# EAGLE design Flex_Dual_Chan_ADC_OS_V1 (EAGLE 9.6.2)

## Sheet 1 of 3: ADC, FE, and Vref
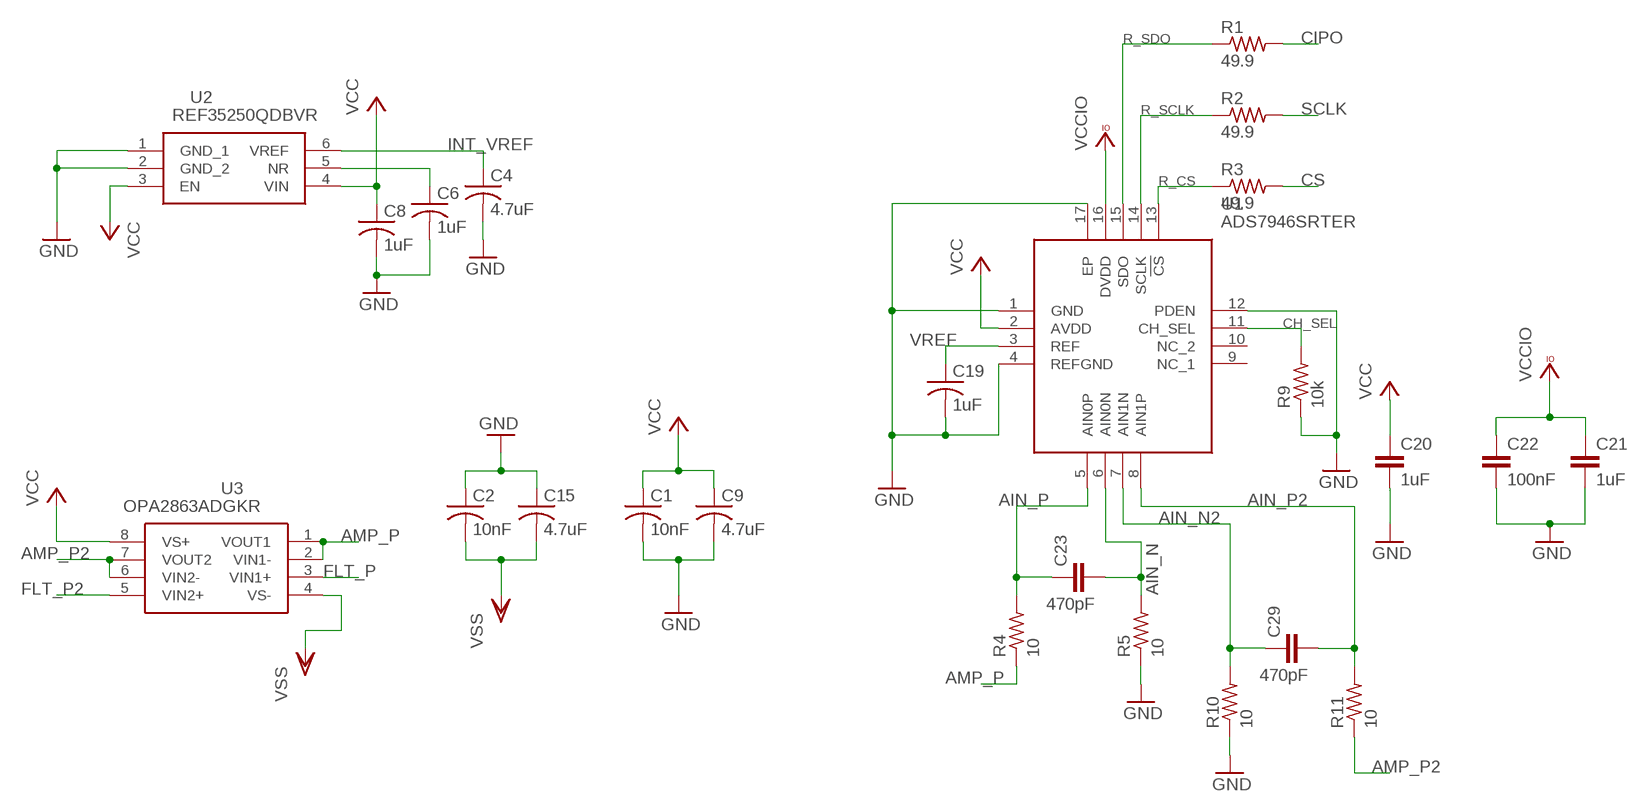
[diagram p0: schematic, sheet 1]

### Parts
C1  10nF  C-USC0603  [C0603]
C2  10nF  C-USC0603  [C0603]
C4  4.7uF  C-USC0603  [C0603]
C6  1uF  C-USC0603  [C0603]
C8  1uF  C-USC0603  [C0603]
C9  4.7uF  C-USC0603  [C0603]
C15  4.7uF  C-USC0603  [C0603]
C19  1uF  C-USC0603  [C0603]
C20  1uF  C-EUC0603  [C0603]
C21  1uF  C-EUC0603  [C0603]
C22  100nF  C-EUC0603  [C0603]
C23  470pF  C-EUC0603  [C0603]
C29  470pF  C-EUC0603  [C0603]
R1  49.9  R-US_R0603  [R0603]
R2  49.9  R-US_R0603  [R0603]
R3  49.9  R-US_R0603  [R0603]
R4  10  R-US_R0603  [R0603]
R5  10  R-US_R0603  [R0603]
R9  10k  R-US_R0603  [R0603]
R10  10  R-US_R0603  [R0603]
R11  10  R-US_R0603  [R0603]
U1  ADS7946SRTER  [QFN50P300X300X80-17N]
U2  REF35250QDBVR  REF35205QDBVR  [SOT95P280X145-6N]
U3  OPA2863ADGKR  [SOP65P490X110-8N]

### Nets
AIN_N: C23.2 R5.2 U1.6(AIN0N)
AIN_N2: C29.1 R10.2 U1.7(AIN1N)
AIN_P: C23.1 R4.2 U1.5(AIN0P)
AIN_P2: C29.2 R11.2 U1.8(AIN1P)
AMP_P: R4.1 U3.1(VOUT1) U3.2(VIN1-)
AMP_P2: R11.1 U3.6(VIN2-) U3.7(VOUT2)
CH_SEL: R9.2 U1.11(CH_SEL) ; also sheet 3
CIPO: R1.2 ; also sheet 3
CS: R3.2 ; also sheet 3
FLT_P: U3.3(VIN1+) ; also sheet 3
FLT_P2: U3.5(VIN2+) ; also sheet 3
GND: C1.2 C2.1 C4.2 C6.2 C8.2 C9.2 C15.1 C19.2 C20.2 C21.2 C22.2 R5.1 R9.1 R10.1 U1.1(GND) U1.4(REFGND) U1.12(PDEN) U1.17(EP) U2.1(GND_1) U2.2(GND_2) ; also sheet 2,3
INT_VREF: C4.1 U2.6(VREF) ; also sheet 2
N$2: C6.1 U2.5(NR)
R_CS: R3.1 U1.13(!CS)
R_SCLK: R2.1 U1.14(SCLK)
R_SDO: R1.1 U1.15(SDO)
SCLK: R2.2 ; also sheet 3
VCC: C1.1 C8.1 C9.1 C20.1 U1.2(AVDD) U2.3(EN) U2.4(VIN) U3.8(VS+) ; also sheet 2
VCCIO: C21.1 C22.1 U1.16(DVDD) ; also sheet 2
VREF: C19.1 U1.3(REF) ; also sheet 2,3
VSS: C2.2 C15.2 U3.4(VS-) ; also sheet 2
Unconnected: U1.9(NC_1) U1.10(NC_2)

## Sheet 2 of 3: Power Circuits
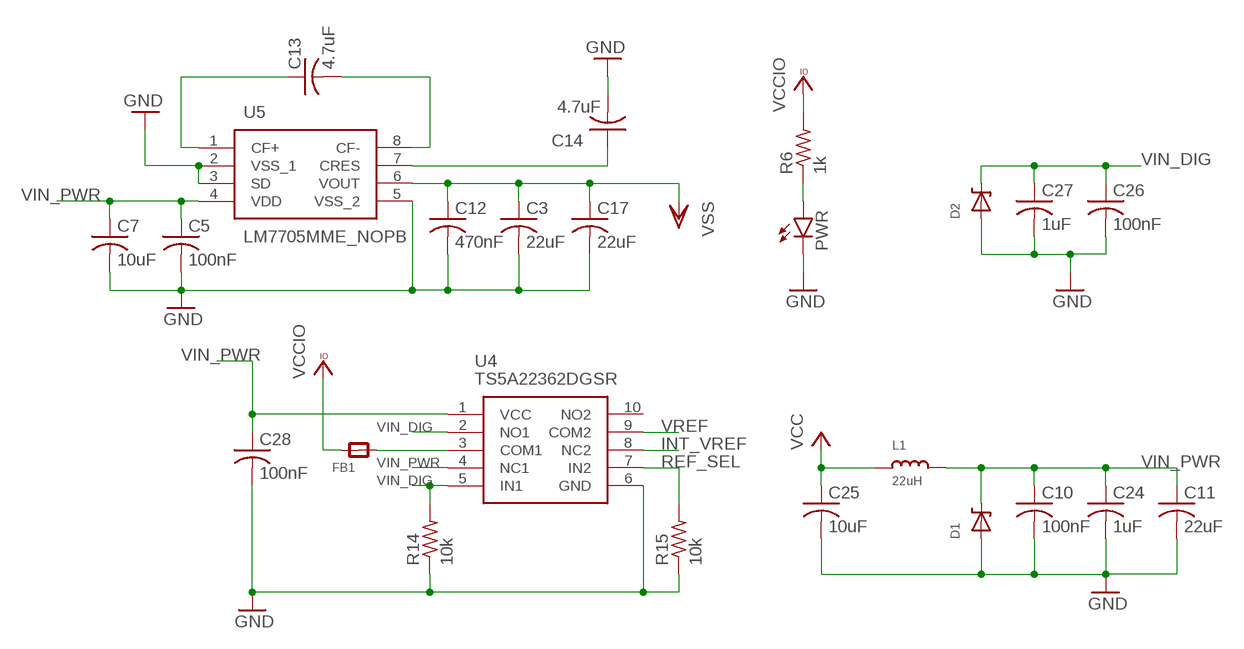
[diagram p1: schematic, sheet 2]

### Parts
C3  22uF  C-USC0603  [C0603]
C5  100nF  C-USC0603  [C0603]
C7  10uF  C-USC0603  [C0603]
C10  100nF  C-USC0603  [C0603]
C11  22uF  C-USC0603  [C0603]
C12  470nF  C-USC0603  [C0603]
C13  4.7uF  C-USC0603  [C0603]
C14  4.7uF  C-USC0603  [C0603]
C17  22uF  C-USC0603  [C0603]
C24  1uF  C-USC0603  [C0603]
C25  10uF  C-USC0603  [C0603]
C26  100nF  C-USC0603  [C0603]
C27  1uF  C-USC0603  [C0603]
C28  100nF  C-USC0603  [C0603]
D1  DDZ5V6ASF  [DDZ5V6ASF]
D2  DDZ5V6ASF  [DDZ5V6ASF]
FB1  FERRITE_0603  [_0603]
L1  22uH  INDUCTOR0805  [0805]
PWR  LEDCHIP-LED0603  [CHIP-LED0603]
R6  1k  R-US_R0603  [R0603]
R14  10k  R-US_R0603  [R0603]
R15  10k  R-US_R0603  [R0603]
U4  TS5A22362DGSR  [SOP50P490X110-10N]
U5  LM7705MME_NOPB  [SOP65P490X110-8N]

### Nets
GND: C3.2 C5.2 C7.2 C10.2 C11.2 C12.2 C14.2 C17.2 C24.2 C25.2 C26.2 C27.2 C28.2 D1.P$1(A) D2.P$1(A) PWR.C R14.1 R15.1 U4.6(GND) U5.2(VSS_1) U5.3(SD) U5.5(VSS_2) ; also sheet 1,3
INT_VREF: U4.8(NC2) ; also sheet 1
N$3: C13.1 U5.1(CF+)
N$4: PWR.A R6.1
N$5: C13.2 U5.8(CF-)
N$6: C14.1 U5.7(CRES)
N$7: FB1.2 U4.3(COM1)
REF_SEL: R15.2 U4.7(IN2)
VCC: C25.1 L1.1 ; also sheet 1
VCCIO: FB1.1 R6.2 ; also sheet 1
VIN_DIG: C26.1 C27.1 D2.P$2(C) R14.2 U4.2(NO1) U4.5(IN1) ; also sheet 3
VIN_PWR: C5.1 C7.1 C10.1 C11.1 C24.1 C28.1 D1.P$2(C) L1.2 U4.1(VCC) U4.4(NC1) U5.4(VDD) ; also sheet 3
VREF: U4.9(COM2) ; also sheet 1,3
VSS: C3.1 C12.1 C17.1 U5.6(VOUT) ; also sheet 1
Unconnected: U4.10(NO2)

## Sheet 3 of 3: Input Filter and Connections
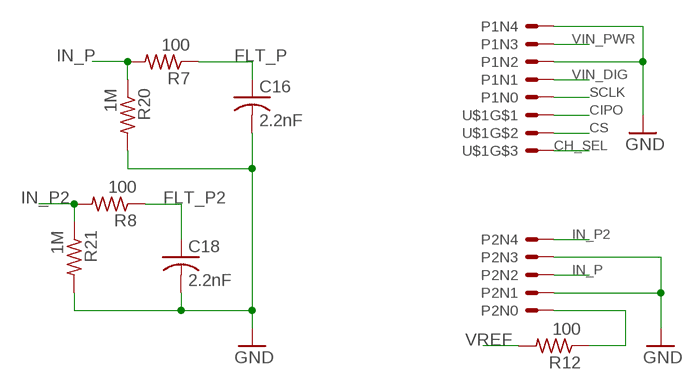
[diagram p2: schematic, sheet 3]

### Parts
C16  2.2nF  C-USC0603  [C0603]
C18  2.2nF  C-USC0603  [C0603]
P1  5PINHEADER  [5PINHEADER]
P2  5PINHEADER  [5PINHEADER]
R7  100  R-US_R0603  [R0603]
R8  100  R-US_R0603  [R0603]
R12  100  R-US_R0603  [R0603]
R20  1M  R-US_R0603  [R0603]
R21  1M  R-US_R0603  [R0603]
U$1  3PINHEADER  [3PINHEADER]

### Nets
CH_SEL: U$1.N2 ; also sheet 1
CIPO: U$1.N0 ; also sheet 1
CS: U$1.N1 ; also sheet 1
FLT_P: C16.1 R7.1 ; also sheet 1
FLT_P2: C18.1 R8.1 ; also sheet 1
GND: C16.2 C18.2 P1.N2 P1.N4 P2.N1 P2.N3 R20.2 R21.2 ; also sheet 1,2
IN_P: P2.N2 R7.2 R20.1
IN_P2: P2.N4 R8.2 R21.1
N$1: P2.N0 R12.1
SCLK: P1.N0 ; also sheet 1
VIN_DIG: P1.N1 ; also sheet 2
VIN_PWR: P1.N3 ; also sheet 2
VREF: R12.2 ; also sheet 1,2

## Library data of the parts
C1-C19 C24-C28 = rcl:C-US: CAPACITOR, American symbol; SPICEPREFIX: C
C20-C23 C29 = rcl:C-EU: CAPACITOR, European symbol; SPICEPREFIX: C
D1 D2 = ForceTronics:DDZ5V6ASF: DDZ5V6ASF 5.42 Zener Diode
FB1 = microbuilder:FERRITE: Ferrite Bead
L1 = microbuilder:INDUCTOR: Inductors
P1 = ForceTronics:5PINHEADER
P2 = ForceTronics-ForceTronics:5PINHEADER
PWR = led:LED: LED
R1-R12 R14 R15 R20 R21 = rcl:R-US_: RESISTOR, American symbol; SPICEPREFIX: R
U1 = SamacSys_Parts:ADS7946SRTER: 14-Bit, 2MSPS, Dual-Channel, Unipolar, Pseudo-Differential, u-Power SAR ADC Source: Datasheet; DESCRIPTION: 14-Bit, 2MSPS, Dual-Channel, Unipolar, Pseudo-Differential, u-Power SAR ADC; HEIGHT: 0.8mm; MANUFACTURER_NAME: Texas Instruments; MANUFACTURER_PART_NUMBER: ADS7946SRTER; MOUSER_PART_NUMBER: 595-ADS7946SRTER; MOUSER_PRICE-STOCK: https://www.mouser.co.uk/ProductDetail/Texas-Instruments/ADS7946SRTER?qs=UlfnwZ2x8nQ8ZHHj9riOig%3D%3D
U2 = SamacSys_Parts:REF35205QDBVR: Voltage References 650-nA quiescent current, 12-ppm/C drift, ultra-low-power precision voltage reference Source: Datasheet; DESCRIPTION: Voltage References 650-nA quiescent current, 12-ppm/C drift, ultra-low-power precision voltage reference; HEIGHT: 1.45mm; MANUFACTURER_NAME: Texas Instruments; MANUFACTURER_PART_NUMBER: REF35205QDBVR; MOUSER_PART_NUMBER: 595-REF35205QDBVR; MOUSER_PRICE-STOCK: https://www.mouser.co.uk/ProductDetail/Texas-Instruments/REF35205QDBVR?qs=rQFj71Wb1eUmjih2GyUdJQ%3D%3D
U3 = SamacSys_Parts:OPA2863ADGKR: Precision Amplifiers Dual, high-precision, low-power, 105MHz, 12V RRIO voltage-feedback amplifier Source: Datasheet; DESCRIPTION: Precision Amplifiers Dual, high-precision, low-power, 105MHz, 12V RRIO voltage-feedback amplifier; HEIGHT: 1.1mm; MANUFACTURER_NAME: Texas Instruments; MANUFACTURER_PART_NUMBER: OPA2863ADGKR
U4 = SamacSys_Parts:TS5A22362DGSR: Texas Instruments TS5A22362DGSR, Analogue Switch Dual SPDT, 2.3 5.5 V, 10-Pin VSSOP Source: Datasheet; DESCRIPTION: Texas Instruments TS5A22362DGSR, Analogue Switch Dual SPDT, 2.3 5.5 V, 10-Pin VSSOP; HEIGHT: 1.1mm; MANUFACTURER_NAME: Texas Instruments; MANUFACTURER_PART_NUMBER: TS5A22362DGSR; MOUSER_PART_NUMBER: 595-TS5A22362DGSR; MOUSER_PRICE-STOCK: https://www.mouser.co.uk/ProductDetail/Texas-Instruments/TS5A22362DGSR?qs=snW7ThfrdqwrWVQhLBj0GQ%3D%3D
U5 = SamacSys_Parts:LM7705MME_NOPB: Texas Instruments LM7705MME/NOPB Inverter, 3 5.25 V, 8-Pin MSOP Source: Datasheet; DESCRIPTION: Texas Instruments LM7705MME/NOPB Inverter, 3 5.25 V, 8-Pin MSOP; HEIGHT: 1.1mm; MANUFACTURER_NAME: Texas Instruments; MANUFACTURER_PART_NUMBER: LM7705MME/NOPB; MOUSER_PART_NUMBER: 926-LM7705MME/NOPB; MOUSER_PRICE-STOCK: https://www.mouser.co.uk/ProductDetail/Texas-Instruments/LM7705MME-NOPB?qs=QbsRYf82W3FggmdQUdGwaQ%3D%3D
U$1 = ForceTronics:3PINHEADER: 3 pin header with oval copper

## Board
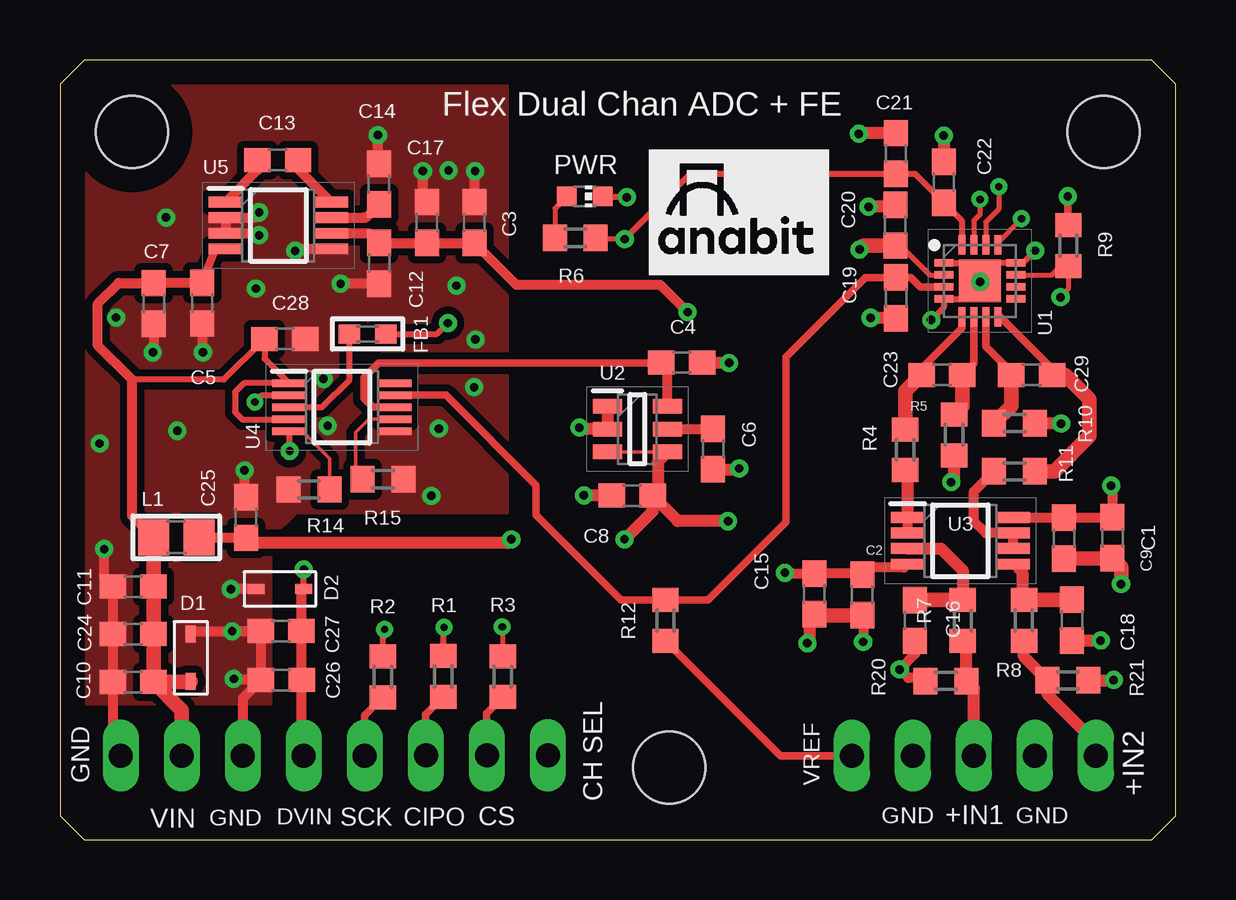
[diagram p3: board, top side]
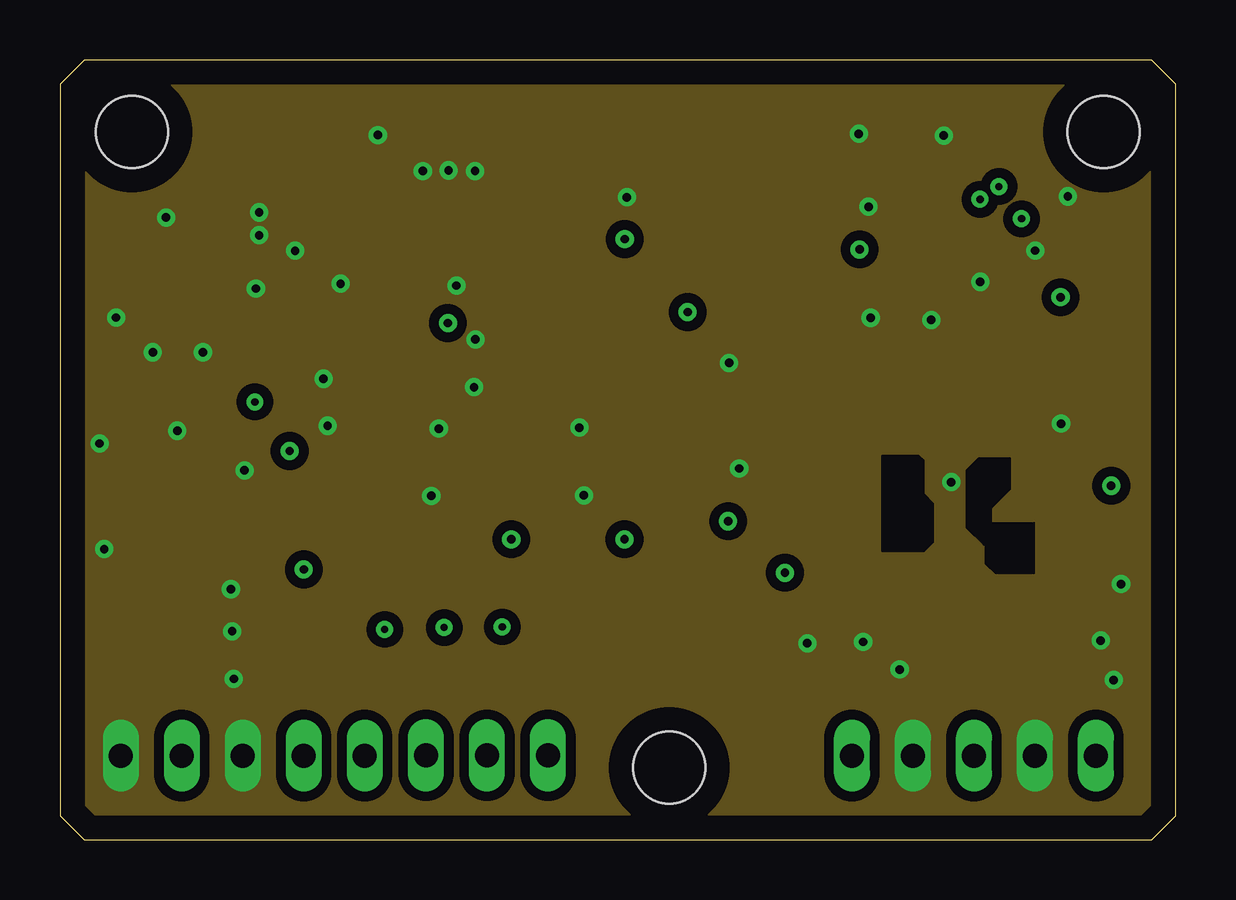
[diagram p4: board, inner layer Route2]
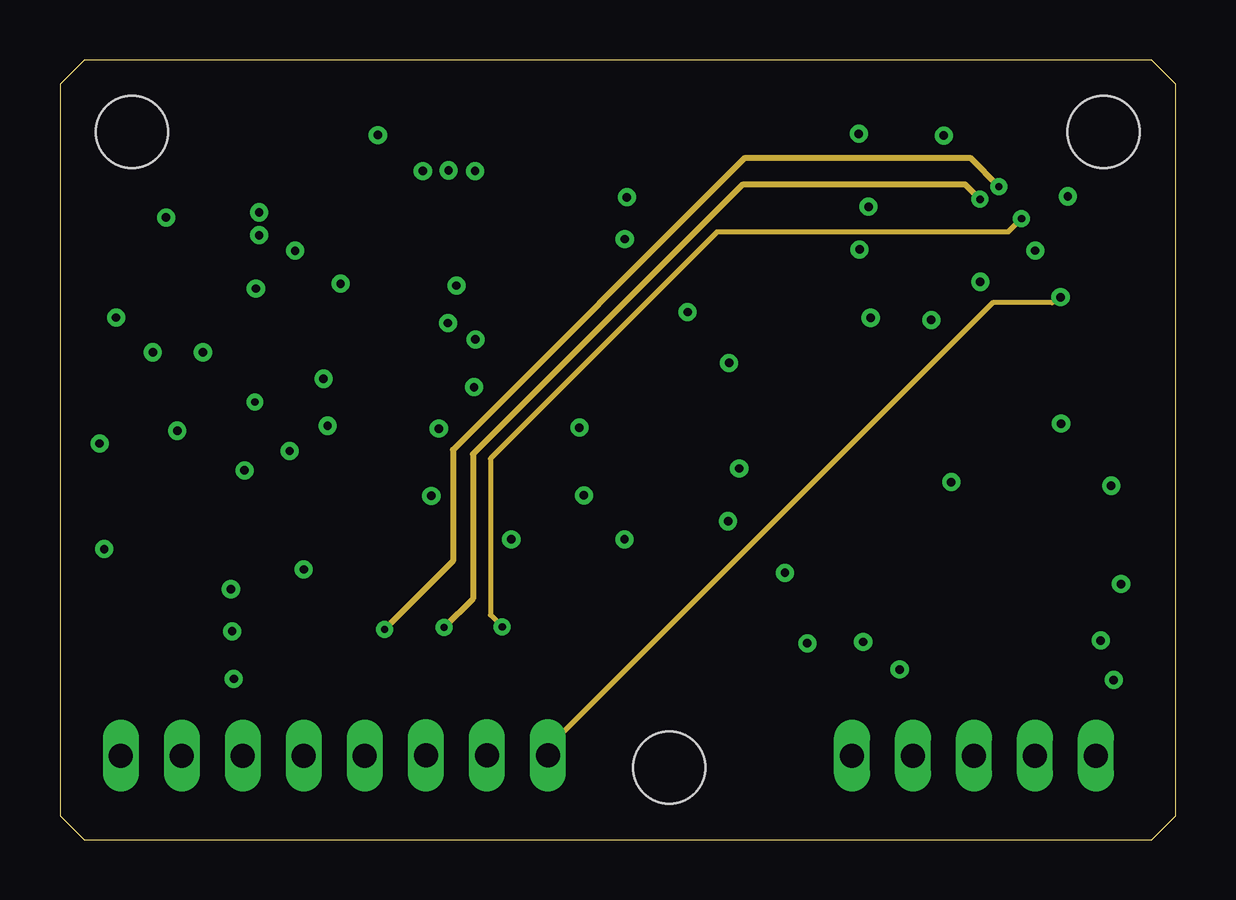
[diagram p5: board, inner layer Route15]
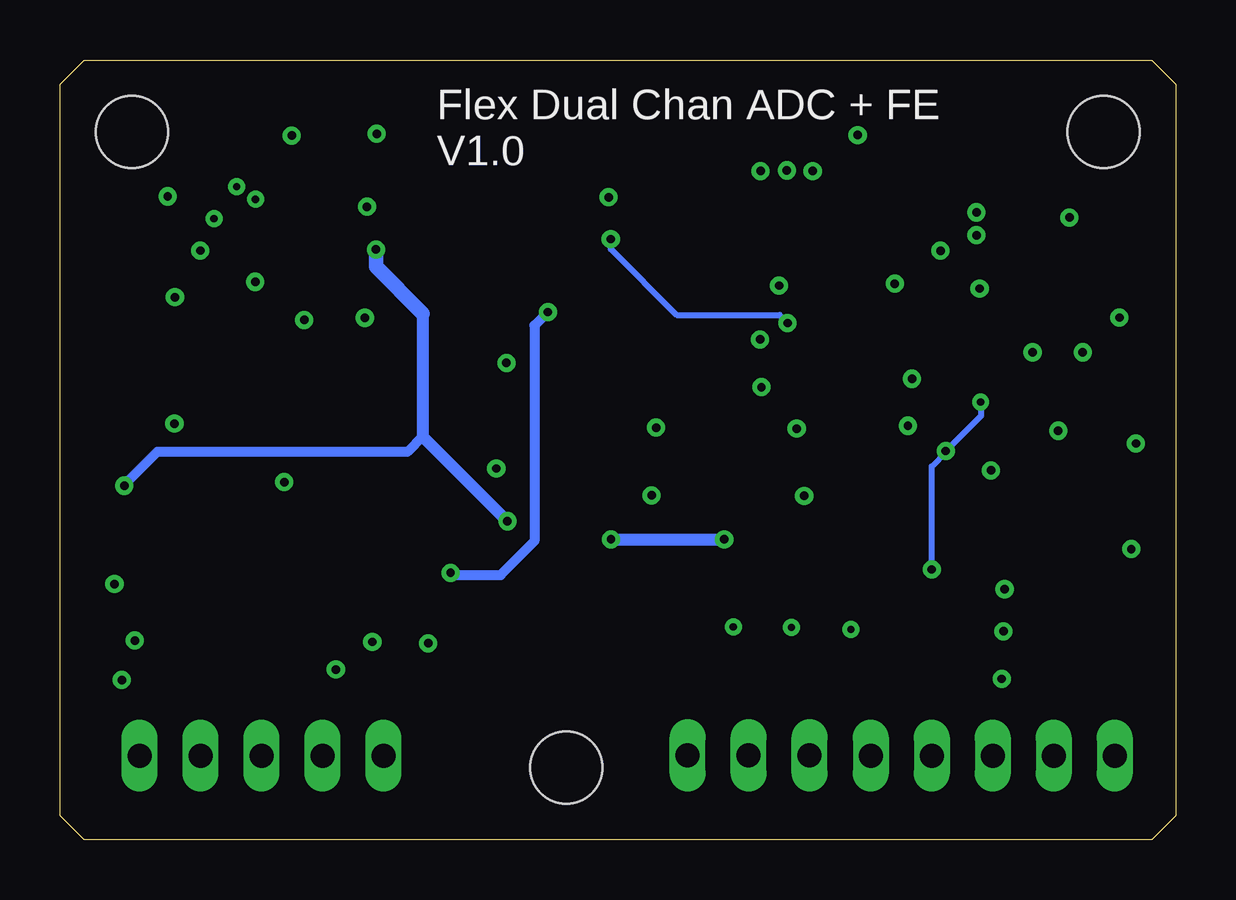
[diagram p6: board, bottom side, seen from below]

Size 46.5 x 32.5 mm. Coordinates in mm from the lower left corner, seen from the top.
Outline: 46.5,1 46.5,31.5 45.5,32.5 1,32.5 0,31.5 0,1 1,0 45.5,0 46.5,1
Copper layers (1*2+15*16): Top 0.035mm / dielectric 0.3mm / Route2 0.035mm / dielectric 1mm / Route15 0.035mm / dielectric 0.3mm / Bottom 0.035mm
Design rules "default *": minimum track width 6mil, minimum drill 0.3mm, track to track 6mil, track to pad 6mil, pad to pad 6mil, via to via 6mil, smd to smd 6mil, copper to edge 40mil, drill to drill 6mil, minimum pad ring 10mil, minimum via ring 8mil, stop-mask expansion 4mil, vias tented up to drill 0mil, thermal gap 10mil
Holes 3 mm at 25.4,3 3,29.5 43.5,29.5

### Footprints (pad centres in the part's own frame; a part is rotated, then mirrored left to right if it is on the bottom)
C0603 = smd 1.1 x 1: 1 -0.85,0; 2 0.85,0
DDZ5V6ASF = smd 0.71 x 0.41: P$1 0,0; P$2 1.99,0
_0603 = smd 0.9 x 0.8: 1 -0.762,0; 2 0.762,0
0805 = smd 1.3 x 1.5: 1 -0.95,0; 2 0.95,0
5PINHEADER = drill 1 long: N0 -5.08,0; N1 -2.54,0; N2 0,0; N3 2.54,0; N4 5.08,0
CHIP-LED0603 = smd 0.8 x 0.8: A 0,-0.75; C 0,0.75
R0603 = smd 1 x 1.1: 1 -0.85,0; 2 0.85,0
QFN50P300X300X80-17N = smd 0.8 x 0.3: 1 -1.5,0.75; 2 -1.5,0.25; 3 -1.5,-0.25; 4 -1.5,-0.75; 9 1.5,-0.75; 10 1.5,-0.25; 11 1.5,0.25; 12 1.5,0.75 | smd 0.3 x 0.8: 5 -0.75,-1.5; 6 -0.25,-1.5; 7 0.25,-1.5; 8 0.75,-1.5; 13 0.75,1.5; 14 0.25,1.5; 15 -0.25,1.5; 16 -0.75,1.5 | smd 1.76 x 1.76: 17 0,0
SOT95P280X145-6N = smd 1.2 x 0.6: 1 -1.25,0.95; 2 -1.25,0; 3 -1.25,-0.95; 4 1.25,-0.95; 5 1.25,0; 6 1.25,0.95
SOP65P490X110-8N = smd 1.4 x 0.45: 1 -2.2,0.975; 2 -2.2,0.325; 3 -2.2,-0.325; 4 -2.2,-0.975; 5 2.2,-0.975; 6 2.2,-0.325; 7 2.2,0.325; 8 2.2,0.975
SOP50P490X110-10N = smd 1.4 x 0.3: 1 -2.2,1; 2 -2.2,0.5; 3 -2.2,0; 4 -2.2,-0.5; 5 -2.2,-1; 6 2.2,-1; 7 2.2,-0.5; 8 2.2,0; 9 2.2,0.5; 10 2.2,1
3PINHEADER = drill 1 long: N0 1.27,1.27; N1 3.81,1.27; N2 6.35,1.27

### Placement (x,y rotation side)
C1  43.86,12.58 270 top
C2  33.44,10.2 90 top
C3  17.27,25.73 90 top
C4  25.92,19.88 0 top
C5  5.92,22.36 270 top
C6  27.22,16.28 270 top
C7  3.91,22.35 270 top
C8  23.85,14.34 180 top
C9  41.84,12.56 270 top
C10  3.05,6.58 180 top
C11  3.05,10.55 180 top
C12  13.3,24.02 270 top
C13  9.07,28.32 0 top
C14  13.3,27.32 90 top
C15  31.45,10.24 90 top
C16  35.64,9.13 270 top
C17  15.3,25.73 90 top
C18  42.18,9.15 270 top
C19  34.84,22.58 270 top
C20  34.82,25.61 90 top
C21  34.85,28.6 90 top
C22  36.85,27.4 90 top
C23  36.76,19.37 0 top
C24  3.05,8.57 180 top
C25  7.75,13.43 90 top
C26  9.22,6.65 180 top
C27  9.22,8.7 180 top
C28  9.38,20.88 0 top
C29  40.5,19.36 0 top
D1  5.45,8.57 270 top
D2  8.18,10.45 0 top
FB1  12.82,21.07 180 top
L1  4.85,12.6 180 top
P1  7.62,3.5 180 top
P2  38.1,3.5 0 top
PWR  21.88,26.81 270 top
R1  15.98,6.8 270 top
R2  13.46,6.78 270 top
R3  18.46,6.79 270 top
R4  35.23,16.25 90 top
R5  37.27,16.87 90 top
R6  21.48,25.09 0 top
R7  37.63,9.13 270 top
R8  40.18,9.14 270 top
R9  42.03,24.76 270 top
R10  39.78,17.36 180 top
R11  39.78,15.35 0 top
R12  25.24,9.14 90 top
R14  10.38,14.6 0 top
R15  13.47,15.02 180 top
R20  36.93,6.61 180 top
R21  42.01,6.64 0 top
U1  38.34,23.29 0 top
U2  24.07,17.11 0 top
U3  37.53,12.46 0 top
U4  11.75,18.02 0 top
U5  9.1,25.6 0 top
U$1  13.99,2.24 0 top

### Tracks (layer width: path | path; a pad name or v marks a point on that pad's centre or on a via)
AIN_N
  Top 0.305: C23.2 38.09,19.85 U1.6
  Top 0.61: R5.2 37.61,18.06 C23.2
AIN_N2
  Top 0.305: U1.7 38.59,20.56 39.65,19.5 C29.1
  Top 0.61: R10.2 39.65,18.08 C29.1
AIN_P
  Top 0.305: U1.5 37.59,21.32 35.87,19.6 35.87,19.33
  Top 0.406: 35.87,19.33 C23.1
  Top 0.61: R4.2 35.23,18.69 35.87,19.33
AIN_P2
  Top 0.305: U1.8 39.19,21.79 41.35,19.63 C29.2
  Top 0.61: R11.2 41.44,15.35 42.91,16.82 42.91,18.36 41.91,19.36 C29.2
AMP_P
  Top 0.406: U3.2 U3.1
  Top 0.508: U3.1 35.34,15.29 R4.1
AMP_P2
  Top 0.406: U3.6 U3.7 38.59,12.78 38.1,13.27 38.1,14.52 R11.1
CH_SEL  (via drill 0.35)
  Top 0.2: 41.75,23.94 41.94,24.12 41.94,24 R9.2 42.03,22.96 41.71,22.64 v41.71,22.61
  Top 0.203: U1.11 41.35,23.54 41.94,24.12
  Route15 0.2: v41.71,22.61 41.59,22.61 41.36,22.38 38.88,22.38 20.34,3.84 U$1.N2
CIPO
  Top 0.305: R1.2 15.24,5.21 15.24,3.53 U$1.N0
CS
  Top 0.305: R3.2 17.78,5.26 17.78,3.53 U$1.N1
FLT_P
  Top 0.508: U3.3 36.72,12.13 37.63,11.22 R7.1
  Top 0.61: R7.1 C16.1
FLT_P2
  Top 0.406: 40.12,11.1 U3.5
  Top 0.508: 40.12,11.1 40.12,10.05 R8.1
  Top 0.61: C18.1 R8.1
GND  (via drill 0.35)
  Top 0.254: v23.63,26.77 23.63,26.81 PWR.C | v40.65,24.55 40.14,24.04 U1.12 39.09,24.04 38.4,23.35 | 38.4,23.35 U1.17 | v36.32,21.66 36.84,22.18 U1.4 37.65,22.54 v38.36,23.25 | U1.1 37.71,24.04 38.4,23.35
  Top 0.305: v42.01,26.81 42.01,25.63 R9.1
  Top 0.406: C14.2 13.25,28.23 v13.25,29.37 | C17.2 15.12,26.75 v15.12,27.87 | C3.2 17.27,27.84 v17.3,27.87 | C12.2 v11.71,23.18 v11.7,23.17 | U5.5 9.88,24.62 v9.8,24.55 | v8.3,26.14 8.08,25.93 U5.2 U5.3 8.22,25.27 v8.3,25.2 | C25.2 7.7,14.33 v7.7,15.39 | v1.84,12.11 1.84,10.9 C11.2 C24.2 C10.2 2.2,3.84 P1.N4 | D1.P$1 5.55,8.68 v7.17,8.68 8.35,8.68 C27.2 C26.2 | D2.P$1 7.13,10.45 v7.12,10.44 | C26.2 7.29,6.65 v7.25,6.7 | C26.2 7.62,5.89 P1.N2 | C7.2 3.91,20.36 v3.87,20.32 | C5.2 5.92,20.35 v5.96,20.31 | R20.2 35.96,6.73 35.36,6.73 v35,7.09 35.64,7.73 C16.2 | C2.1 33.48,9.31 v33.48,8.24
  Top 0.508: C6.2 28.27,15.43 v28.31,15.47 | C8.2 v21.85,14.34 v21.84,14.35 | U2.1 U2.2 21.71,17.11 v21.65,17.17 | v27.89,19.87 C4.2 | C19.2 33.81,21.73 v33.79,21.75 | C20.2 34.74,26.38 v33.7,26.38 | C21.2 33.33,29.45 v33.3,29.42 | v36.84,29.35 C22.2 | R10.1 41.71,17.36 v41.73,17.34 | R5.1 37.27,15.02 v37.15,14.9 | C15.1 31.24,9.18 31.24,8.23 31.2,8.23 v31.15,8.18 | C18.2 v43.38,8.3 | R21.2 v43.91,6.64 v43.92,6.65
  Top 0.61: C9.2 43.84,11.71 C1.2 44.23,11.36 v44.23,10.65 | C18.2 42.27,8.3 | C2.1 31.49,9.35 C15.1
  other vias: 8.16,22.97 16.52,23.09 16.2,27.89 2.34,21.76 10.98,19.21 11.15,17.25 4.89,17.04 15.48,14.33 4.42,25.93 17.32,20.85 1.65,16.51 17.26,18.86 15.79,17.13
  pour Route2 (isolate 0.406, no thermals): -3,-1 -3,37 50,37 50,-2 -2,-2
  pour Top (isolate 0.305, no thermals): -1.25,5.64 8.83,5.64 8.83,12.58 9.88,13.62 18.68,13.62 18.68,31.82 15.75,34.75 -1.25,34.75
  cutout Route2: 35.8,16 34.27,16 34.27,12.03 36.03,12.03 36.4,12.4 36.4,14 36,14.4 36,15.8
  cutout Route2: 40.6,11.1 39,11.1 38.6,11.5 38.6,12.3 38.5,12.3 37.8,13 37.8,15.4 38.3,15.9 39.6,15.9 39.6,14.6 38.8,13.8 38.8,13.2 40.6,13.2
IN_P
  Top 0.508: P2.N2 38.1,6.29 R20.1 37.78,8.13 R7.2
IN_P2
  Top 0.508: P2.N4 43.18,4.04 41.16,6.06 R21.1 40.18,7.62 R8.2
INT_VREF
  Top 0.305: U4.8 13.04,18.02 12.68,18.39 12.68,19.25 13.29,19.87 C4.1
  Top 0.406: U2.6 25.32,19.63 C4.1
N$1
  Top 0.305: R12.1 30.03,3.5 P2.N0
N$2
  Top 0.406: U2.5 26.79,17.11 C6.1
N$3
  Top 0.406: U5.1 8.22,27.9 C13.1
N$4
  Top 0.2: PWR.A 20.62,26.31 R6.1
N$5
  Top 0.406: C13.2 9.93,27.95 U5.8
N$6
  Top 0.406: U5.7 12.65,25.93 12.76,25.93 C14.1
N$7
  Top 0.254: U4.3 10.93,18.02 12.06,19.16 FB1.2
R_CS  (via drill 0.3)
  Top 0.203: R3.1 18.46,8.84 v18.43,8.87 | v40.08,25.87 v40.08,25.88 39.09,24.89 U1.13
  Route15 0.203: v18.43,8.87 17.95,9.36 17.95,15.88 27.41,25.34 39.54,25.34 v40.08,25.88
R_SCLK  (via drill 0.3)
  Top 0.2: R2.1 13.46,7.78
  Top 0.203: v39.14,27.22 39.14,26.29 38.59,25.74 U1.14
  Top 0.254: v13.54,8.76 13.46,8.69 R2.1
  Route15 0.254: v13.54,8.76 16.38,11.61 16.38,16.25 28.55,28.42 37.94,28.42 v39.14,27.22
R_SDO  (via drill 0.3)
  Top 0.203: v38.35,26.69 38.35,26.06 38.09,25.8 U1.15
  Top 0.254: R1.1 15.98,8.84 v16.02,8.84 | v38.35,26.69 38.38,26.66
  Route15 0.254: v16.02,8.84 17.21,10.04 17.21,16.07 28.47,27.32 37.72,27.32 v38.35,26.69
REF_SEL
  Top 0.152: U4.7 12.88,17.52 12.33,16.97 12.33,15.31 R15.2
SCLK
  Top 0.305: P1.N0 12.7,5.17 R2.2
VCC  (via drill 0.35)
  Top 0.152: U2.3 U2.4
  Top 0.203: C20.1 35.04,24.76 36.26,23.54 U1.2
  Top 0.254: v33.33,24.6 33.49,24.76
  Top 0.305: v27.85,13.28 v27.85,13.27
  Top 0.406: 24.74,14.3 C8.1 24.92,14.56 | L1.1 7.72,12.6 C25.1 | v43.82,14.75 43.86,14.71 C1.1 43.84,13.41 C9.1 39.76,13.41 U3.8
  Top 0.508: 24.92,14.56 24.92,15.76 U2.4 | C25.1 7.97,12.36 18.65,12.36 v18.81,12.52 | v23.53,12.52 24.7,13.69 C8.1 25.76,13.28 v27.85,13.28
  Top 0.61: 33.49,24.76 C20.1
  Bottom 0.406: 31.38,16.8 32.02,16.16 42.44,16.16 43.82,14.78 v43.82,14.75
  Bottom 0.508: v23.53,12.52 v18.81,12.52 | v27.85,13.27 31.38,16.8 31.38,21.93
  Bottom 0.61: 31.38,21.93 33.33,23.88 v33.33,24.6
VCCIO  (via drill 0.35)
  Top 0.2: v23.54,25.03 22.38,25.03 R6.2
  Top 0.254: C21.1 35.65,27.75 C22.1 37.59,25.81 U1.16 | C21.1 34.56,27.46 | FB1.1 15.71,21.07 v16.17,21.53 | v23.54,25.03 26.26,27.75 C21.1
  Bottom 0.254: v16.17,21.53 16.51,21.87 20.8,21.87 23.54,24.61 v23.54,25.03
VIN_DIG  (via drill 0.3, 0.35)
  Top 0.152: R14.2 11.23,15.88 10.09,17.02 U4.5
  Top 0.254: D2.P$2 10.16,11.23 v10.15,11.25 v10.16,11.26 | v9.57,16.2 9.57,17 U4.5 | v8.12,18.24 8.41,18.52 U4.2
  Top 0.406: P1.N1 10.07,3.58 C26.1 C27.1 10.07,10.36 D2.P$2
  Bottom 0.254: v10.16,11.26 10.16,15.56 9.55,16.18 v9.57,16.2 8.1,17.68 8.1,18.24 v8.12,18.24
VIN_PWR
  Top 0.254: 3,19.18 6.83,19.18 C28.1 8.53,20.05 U4.1 7.67,19.02 7.3,18.65 7.3,17.82 7.62,17.5 9.53,17.5 U4.4
  Top 0.305: C5.1 6.46,24.62
  Top 0.406: L1.2 3,13.5 3,19.18 1.58,20.59 1.58,22.34 2.44,23.2 C7.1 C5.1 | 6.46,24.62 U5.4
  Top 0.61: P1.N3 5.08,5.39 C10.1 | C10.1 D1.P$2 | C10.1 C24.1 C11.1 L1.2
VREF
  Top 0.203: U1.3
  Top 0.305: C19.1 34.99,23.43 34.97,23.41 | C19.1 35.46,23.43 35.86,23.03 U1.3 | U4.9 16.09,18.52 19.84,14.77 19.84,13.54 23.39,9.99 R12.2 27.01,9.99 30.25,13.23 30.25,20.11 33.57,23.43 C19.1
VSS  (via drill 0.35)
  Top 0.305: 19.18,23.12 19.03,23.12 | 31.43,11.07 C15.2
  Top 0.406: U5.6 12.9,25.27 C12.1 C17.1 C3.1 19.03,23.12 | v26.16,21.99 25.03,23.12 19.18,23.12 | v30.22,11.12 30.27,11.07 31.43,11.07 | C15.2 33.4,11.09 C2.2 33.73,11.34 35.2,11.34 U3.4
  Bottom 0.406: v26.16,21.99 26.72,21.43 26.72,12.44 28.13,11.03 30.13,11.03 v30.22,11.12

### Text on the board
tNames: Flex Dual Chan ADC + FE | GND | CH SEL | VREF | +IN2 | VIN | GND | DVIN | SCK | CIPO | CS | GND | +IN1 | GND
bNames: Flex Dual Chan ADC + FE / V1.0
